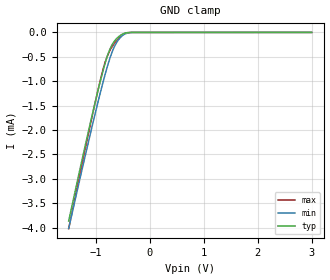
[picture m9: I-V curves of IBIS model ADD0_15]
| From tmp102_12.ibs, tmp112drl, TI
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|   ADD0_15   1.8V digital input Model
[Model] ADD0_15
Model_type   Input
| Signals   ADD0(4)
Vinl = 0.45
Vinh = 1.05
|   typ   min   max
|   (nom PVT)   (Fast PVT)   (slow PVT)
|Average
C_comp   5.9438150e-13 5.8266310e-13 6.0446480e-13
| Where   nom PVT is  Nominal Process, 1.5V, 27C
|   Fast PVT is Strong Process, 1.6V, -40C
|   Slow PVT is Weak Process, 1.4V, 125C
[Voltage Range]   1.5   1.4   1.6
[Temperature Range]   27   125   -40
|Ambient Temperature   27   125   -40
[Power Clamp Reference]   1.5   1.4   1.6
[GND Clamp Reference]   0   0   0
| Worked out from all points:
|   GND clamp passes 1 mA (typ) near -0.91 V on its own axis
[GND Clamp]
|   Voltage   I(typ)   I(min)   I(max)
-1.5V     -3.861mA   -4.014mA   -4.019mA
-1.278V   -2.733mA   -2.928mA   -2.827mA
-1.073V   -1.733mA   -1.956mA   -1.758mA
-944.8mV  -1.135mA   -1.37mA    -1.12mA
-859.1mV  -764.8uA   -999uA     -737.7uA
-792.7mV  -514uA     -731.9uA   -507.7uA
-712.5mV  -286.9uA   -452.2uA   -321.2uA
-624.9mV  -142.6uA   -229.6uA   -181.8uA
-516.2mV  -42.52uA   -76.66uA   -56.11uA
-413.8mV  -5.086uA   -14.06uA   -7.981uA
-283.3mV  -720.1nA   -701.7nA   -385nA
2.995V    0A         0A         0A
[POWER Clamp]
|   SCR cell for ESD function. Effects occurr above VDD x 2
|   Voltage   I(typ)   I(min)   I(max)
-1.5V     0A         0A         0A
0V        0A         0A         0A
3V        0A         0A         0A
